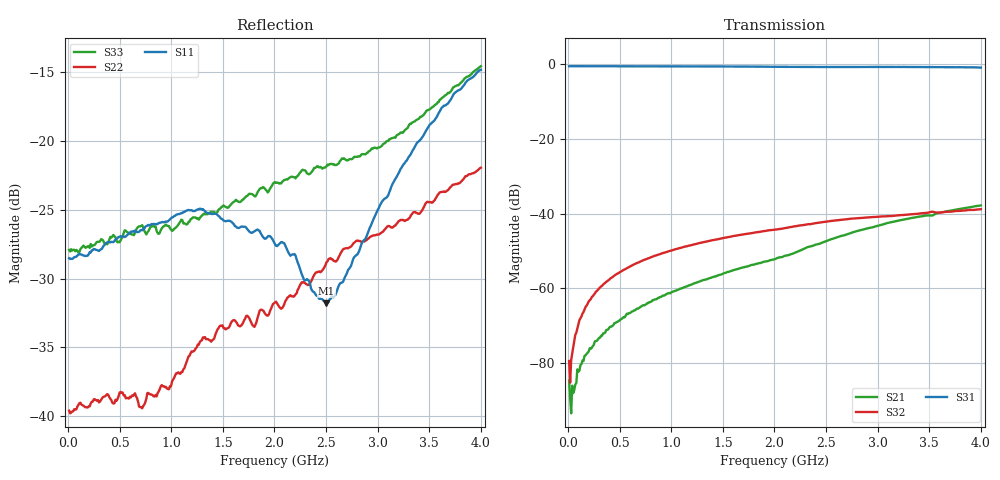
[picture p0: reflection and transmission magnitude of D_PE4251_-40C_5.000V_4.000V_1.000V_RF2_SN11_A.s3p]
! Device ID: PE4251_SoldCshunt_081809
! Dir: c:\Test Bench Repositories\Bench_Software_CVI_Version_8\trunk\PSC 4Port_VNA Bench\datalog\4250\TEST\PE4251_SoldCshunt_081809\-40C\5p000000\RF2
! Serial: 11
! Insertion: A
! Temp: -40C
! VDD: 5.000
! Control_Hi: 80.000
! Control_Lo: 20.000
! Logic State: RF2
! Port 1: RFC
! Port 2: RF1
! Port 3: RF2
! V1 = 1.00
! V2 = 1.00
! V3 = 1.00
! IDD: 5.881870e-05
! FILE NAME
! DATE 08/18/09  20:10
! CORRECTED  DATA
#  Hz  S  RI  R  50.00
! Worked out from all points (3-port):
!   401 points, 10 MHz to 4 GHz, reference 50 ohm
!   strongest paths, dB at 10 MHz, 1.008 GHz, 2.005 GHz, 3.002 GHz, 4 GHz:
!     S31: -0.5, -0.5, -0.6, -0.7, -0.8
!     S32: -79.5, -49.9, -44.3, -40.8, -38.8
!     S21: -84.8, -61.1, -52.2, -43.3, -37.8
!   lowest |S11| = -31.8 dB at 2.504 GHz (marker M1), VSWR 1.05, Z = 50.6 - j2.52 ohm
!   |S11| at or under -10 dB: start of sweep to end of sweep
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1e7  0.0375 -0.000633  5.19e-05 -6.84e-05  0.9436 -0.0035
     5.66e-05 -9.37e-06  0.0105 -0.00073  4.36e-05 4.51e-05
     0.9452 -0.00496  0.0001 3.3e-05  0.0402 0.000581
8.98e7  0.0383 0.0018  8.84e-06 -6.82e-05  0.9456 -0.0324
        2.13e-05 -7.85e-05  0.0108 0.000142  3e-05 0.000301
        0.9467 -0.0326  2.95e-05 0.000287  0.0399 -0.000689
1.696e8  0.038 0.00324  -5.48e-06 -0.000117  0.9428 -0.0597
         -1.18e-05 -0.000125  0.0107 0.00132  4.47e-05 0.000561
         0.9437 -0.0599  2.7e-05 0.000559  0.0408 0.00156
4.888e8  0.0444 0.00545  -0.00019 -0.000317  0.9274 -0.1686
         -0.000178 -0.000314  0.0114 0.00302  0.000151 0.00159
         0.9279 -0.1683  0.000147 0.00158  0.0429 -0.00251
7.18225e8  0.0473 0.0024  -0.00038 -0.000431  0.9101 -0.2447
           -0.000394 -0.000427  0.01 0.00371  0.000284 0.0023
           0.9113 -0.2445  0.000264 0.00232  0.0492 -0.00513
1.2868e9  0.056 -0.00859  -0.00112 -0.000549  0.8372 -0.4227
          -0.00112 -0.000546  0.017 0.00802  0.00071 0.00399
          0.84 -0.4225  0.00071 0.00399  0.0524 -0.0085
2.005e9  0.038 -0.0183  -0.00234 -0.000757  0.7013 -0.6087
         -0.00233 -0.000752  0.0166 0.0199  0.00128 0.00597
         0.7033 -0.6078  0.00128 0.00596  0.0649 -0.0284
2.50375e9  0.00643 -0.0249  -0.00409 -0.00123  0.5906 -0.7076
           -0.00411 -0.00125  0.0185 0.0312  0.00177 0.00758
           0.593 -0.7074  0.00176 0.0076  0.0532 -0.0609
3.371575e9  -0.0895 -0.0373  -0.00895 0.000218  0.3573 -0.8496
            -0.00896 0.000226  -0.000442 0.0548  0.00269 0.00948
            0.3596 -0.8509  0.00267 0.00952  -0.0188 -0.1173
4e9  -0.1798 -0.0219  -0.0126 0.00259  0.136 -0.8978
     -0.0126 0.00258  -0.0293 0.0744  0.00289 0.011
     0.1374 -0.8965  0.00289 0.0111  -0.1283 -0.1356
